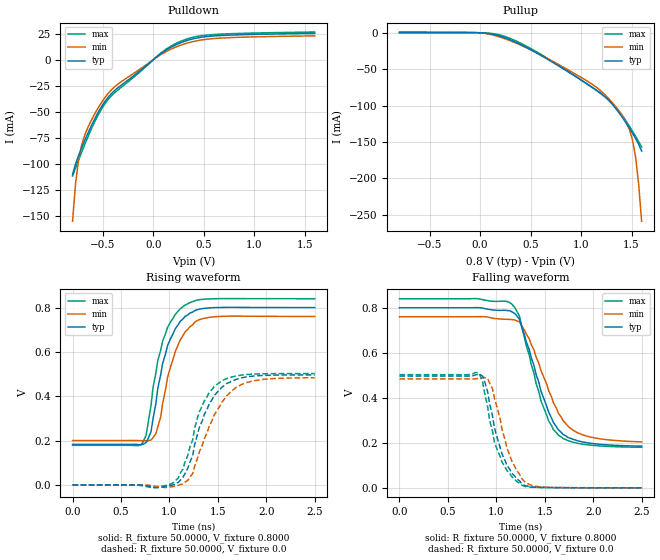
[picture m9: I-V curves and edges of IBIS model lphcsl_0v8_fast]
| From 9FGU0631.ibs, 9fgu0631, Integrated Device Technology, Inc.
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[Model]  lphcsl_0v8_fast
Model_type Output
Polarity   Non-Inverting
Enable   Active-High
Vmeas =  0.4000V
Cref =   2.0000pF
Rref =   0.0
Vref =   0.4000V
C_comp   1.1000pF   1.0000pF   1.2000pF
[Temperature Range]   25.0000   75.0000   0.0
[Voltage Range]   0.8000V   0.7600V   0.8400V
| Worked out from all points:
|   slope of the pulldown table from 0 to 0.12 V, typ, clamps not added: 13.7 ohm
|   slope of the pullup table from 0 to 0.12 V, typ, clamps not added: 63 ohm
|   rising waveform, R_fixture 50.0000, V_fixture 0.8000: 20-80 % time 197ps typ, 194ps min, 186ps max; typ from 0.183 V to 0.8 V
|   rising waveform, R_fixture 50.0000, V_fixture 0.0: 20-80 % time 246ps typ, 296ps min, 234ps max; typ from 0 V to 0.496 V
|   falling waveform, R_fixture 50.0000, V_fixture 0.8000: 20-80 % time 280ps typ, 317ps min, 262ps max; typ from 0.8 V to 0.185 V
|   falling waveform, R_fixture 50.0000, V_fixture 0.0: 20-80 % time 189ps typ, 199ps min, 190ps max; typ from 0.496 V to 0 V
[Pulldown]
|Voltage   I(typ)   I(min)   I(max)
-800mV    -110.2mA   -155mA     -111.5mA
-770mV    -99.93mA   -118.5mA   -103.7mA
-740mV    -91.85mA   -95.72mA   -96.19mA
-710mV    -84.57mA   -81.85mA   -88.81mA
-680mV    -77.65mA   -72.57mA   -81.59mA
-590mV    -58.63mA   -53.65mA   -61.5mA
-500mV    -43.03mA   -39.19mA   -45.27mA
-350mV    -26.89mA   -23.4mA    -29.01mA
100mV     7.489mA    6.294mA    8.221mA
340mV     18.58mA    16.02mA    20.1mA
670mV     23.16mA    20.72mA    24.52mA
1.6V      25.23mA    22.86mA    26.52mA
[Pullup]
|Voltage   I(typ)   I(min)   I(max)
-800mV    337.7uA    1.065mA    85.49uA
-50mV     204.4uA    529.3uA    54.19uA
220mV     -5.557mA   -6.902mA   -3.893mA
580mV     -29.32mA   -28.93mA   -27.89mA
1.15V     -78.54mA   -74.62mA   -79.03mA
1.27V     -92.39mA   -89.84mA   -91.65mA
1.36V     -107mA     -104.8mA   -104.8mA
1.48V     -131.4mA   -133.4mA   -128.6mA
1.51V     -138.1mA   -147.7mA   -135.4mA
1.54V     -145.2mA   -170.8mA   -142.4mA
1.57V     -153mA     -207.1mA   -149.6mA
1.6V      -162.5mA   -259mA     -157mA
[Ramp]
| variable   typ   min   max
dV/dt_r  0.2978/0.2695n   0.2902/0.2963n   0.3015/0.2554n
dV/dt_f  0.3688/0.2750n   0.3334/0.3100n   0.3959/0.2641n
R_load = 50.0000
[Rising Waveform]
R_fixture= 50.0000
V_fixture= 0.8000
V_fixture_min= 0.7600
V_fixture_max= 0.8400
|time   V(typ)   V(min)   V(max)
0s        183.3mV    200.3mV    178.8mV
710ps     181.7mV    200.1mV    182.6mV
760ps     191.7mV    199.1mV    225.6mV
810ps     240.4mV    202.9mV    359mV
860ps     367.1mV    231.4mV    505.2mV
930ps     549.2mV    369.2mV    649.6mV
1.06ns    704.7mV    601.3mV    769.2mV
1.16ns    759.7mV    688.8mV    810.8mV
1.41ns    798.6mV    755.8mV    839mV
2.5ns     800mV      760mV      839.9mV
[Rising Waveform]
R_fixture= 50.0000
V_fixture= 0.0
V_fixture_min= 0.0
V_fixture_max= 0.0
|time   V(typ)   V(min)   V(max)
0s        0V         0V         0V
860ps     -11.54mV   -5.678mV   -11.84mV
1.04ns    716.9uV    -6.959mV   9.755mV
1.14ns    35.12mV    5.063mV    72.51mV
1.24ns    132.8mV    51.7mV     204.4mV
1.31ns    261.3mV    150.8mV    331.1mV
1.49ns    416.6mV    335.6mV    453.5mV
1.64ns    467.9mV    424mV      486.4mV
1.79ns    487mV      461.4mV    497.9mV
2.5ns     496.4mV    483.6mV    502.5mV
[Falling Waveform]
R_fixture= 50.0000
V_fixture= 0.8000
V_fixture_min= 0.7600
V_fixture_max= 0.8400
|time   V(typ)   V(min)   V(max)
0s        800mV      760mV      840mV
1.14ns    786.5mV    748.1mV    822.6mV
1.24ns    748.3mV    737.4mV    761.9mV
1.34ns    614.4mV    661.4mV    589.8mV
1.46ns    430.6mV    521.7mV    387.3mV
1.54ns    336.4mV    431.5mV    297.6mV
1.64ns    257.7mV    332.1mV    233.9mV
1.74ns    223.5mV    273.6mV    209.4mV
1.89ns    203.8mV    235.4mV    194.1mV
2.5ns     185.3mV    204.3mV    180.2mV
[Falling Waveform]
R_fixture= 50.0000
V_fixture= 0.0
V_fixture_min= 0.0
V_fixture_max= 0.0
|time   V(typ)   V(min)   V(max)
0s        496.5mV    483.9mV    502.6mV
810ps     504.4mV    485.9mV    512.8mV
860ps     495.4mV    490.4mV    467.9mV
880ps     471.2mV    489.8mV    420mV
960ps     321.2mV    440.5mV    252.2mV
1.01ns    221mV      353.8mV    168.1mV
1.11ns    99.96mV    176.4mV    76.36mV
1.26ns    19.66mV    42.68mV    12.51mV
1.46ns    1.862mV    4.198mV    1.416mV
2.5ns     50.29uV    92.82uV    34.76uV
